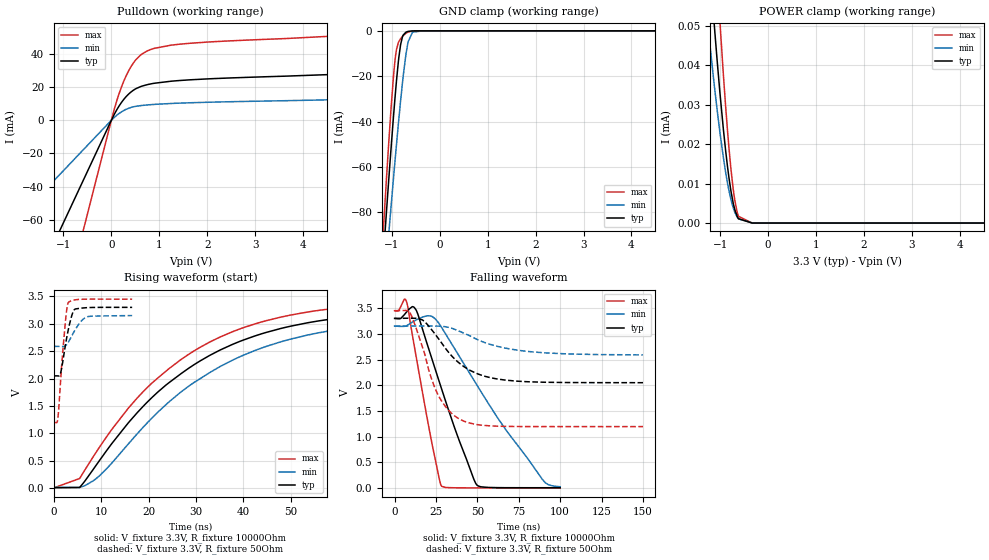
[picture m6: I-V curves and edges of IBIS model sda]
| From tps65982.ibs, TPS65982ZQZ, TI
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|   sda Model
[Model]   sda
Model_type   I/O_open_drain
Polarity   Non-Inverting
Vinl = 0.80
Vinh = 2.00
Vmeas = 1.65
Vref = 3.3
Cref = 2pF
Rref = 10000
|   typ   min   max
|   (nom PVT)   (fast PVT)   (slow PVT)
C_comp   8.631e-13   8.474e-13   8.892e-13
| Where nom  PVT is Nominal Process, 3.3V, 27C
|   Fast PVT is Strong Process,  3.45V, -40C
|   Slow PVT is Weak Process,   3.15V, 125C
[Voltage Range]   3.3   3.15   3.45
|Junction Temperature
[Temperature Range]   27   125   -40
[Pullup Reference]   3.3   3.15   3.45
[Pulldown Reference]   0   0   0
[Power Clamp Reference]   3.3   3.15   3.45
[GND Clamp Reference]   0   0   0
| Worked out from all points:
|   slope of the pulldown table from 0 to 0.495 V, typ, clamps not added: 26.4 ohm
|   GND clamp passes 1 mA (typ) near -0.72 V on its own axis
|   falling waveform, V_fixture 3.3V, R_fixture 10000Ohm: 20-80 % time 20.9ns typ, 38.8ns min, 11.8ns max; typ from 3.3 V to 0.005 V
|   rising waveform, V_fixture 3.3V, R_fixture 10000Ohm: 20-80 % time 26.8ns typ, 28.1ns min, 25.7ns max; typ from 0.005 V to 3.28 V
|   falling waveform, V_fixture 3.3V, R_fixture 50Ohm: 20-80 % time 21.9ns typ, 30.4ns min, 15.2ns max; typ from 3.3 V to 2.05 V
|   rising waveform, V_fixture 3.3V, R_fixture 50Ohm: 20-80 % time 1.6ns typ, 2.37ns min, 1.21ns max; typ from 2.05 V to 3.3 V
[Pulldown]
|   Voltage   I(typ)   I(min)   I(max)
-3.3V     -204.1mA   -100.3mA   -374.1mA
-55.5mV   -3.433mA   -1.687mA   -6.291mA
63.75mV   3.72mA     1.782mA    6.922mA
132.8mV   7.276mA    3.46mA     13.56mA
308.7mV   14.28mA    6.613mA    26.84mA
412.2mV   17.12mA    7.756mA    32.46mA
519.2mV   19.17mA    8.464mA    36.77mA
753.8mV   21.53mA    9.255mA    41.92mA
1.251V    23.57mA    10.13mA    45.33mA
1.645V    24.41mA    10.56mA    46.48mA
5.363V    28.43mA    12.81mA    51.9mA
6.6V      30.96mA    14.1mA     56.05mA
[GND Clamp]
|   Voltage   I(typ)   I(min)   I(max)
-3.3V     -791.8mA   -699.1mA   -889.8mA
-1.224V   -114.3mA   -131mA     -104.8mA
-1.109V   -79.45mA   -101.3mA   -64.81mA
-1.048V   -61.35mA   -85.78mA   -44.54mA
-964.4mV  -38mA      -65.16mA   -20.22mA
-909.2mV  -23.91mA   -51.95mA   -9.276mA
-815.1mV  -6.041mA   -30.79mA   -3.458mA
-704.4mV  -609.6uA   -10.43mA   -1.076mA
-656.7mV  -253.9uA   -4.76mA    -515.7uA
-565.8mV  -41.12uA   -559.3uA   -79.89uA
-330mV    -101.2nA   -940.3nA   -65.96nA
6.6V      0A         0A         0A
[POWER Clamp]
|   Voltage   I(typ)   I(min)   I(max)
-3.3V     548.7uA    403.1uA    721.8uA
-1.299V   79.98uA    55.9uA     116.4uA
-1.208V   64.23uA    44.79uA    94.82uA
-1.111V   48.63uA    33.84uA    73.12uA
-1.004V   33.07uA    23.01uA    51.08uA
-881.5mV  18.07uA    12.69uA    29.13uA
-815.1mV  11.51uA    8.232uA    19.09uA
-774.6mV  8.211uA    6.002uA    13.83uA
-695.3mV  3.499uA    2.796uA    5.93uA
-615.9mV  1.099uA    1.051uA    1.702uA
-330mV    0A         10.54nA    0A
6.6V      0A         0A         0A
[Ramp]
R_load = 10000
|   typ   min   max
dV/dt_r   1.96448/2.68001e-08   1.86582/2.80203e-08   2.05933/2.56579e-08
dV/dt_f   1.97678/2.08968e-08   1.87506/3.88653e-08   2.06819/1.17646e-08
[Falling Waveform]
V_fixture = 3.3V
V_fixture_min = 3.15V
V_fixture_max = 3.45V
R_fixture = 10000Ohm
|   Time   V(typ)   V(min)   V(max)
0s        3.3V       3.15V      3.45V
2.424ns   3.294V     3.145V     3.453V
5.862ns   3.371V     3.145V     3.673V
7.466ns   3.433V     3.162V     3.601V
13.1ns    3.458V     3.27V      2.544V
22.06ns   2.561V     3.344V     951.2mV
28.5ns    1.918V     3.118V     32.31mV
49.65ns   59.37mV    2.006V     3.042mV
89.15ns   5.387mV    171.5mV    3.011mV
100ns     5.367mV    24.9mV     3.011mV
[Rising Waveform]
V_fixture = 3.3V
V_fixture_min = 3.15V
V_fixture_max = 3.45V
R_fixture = 10000Ohm
|   Time   V(typ)   V(min)   V(max)
0s        5.363mV    10.67mV    3.011mV
5.446ns   9.247mV    13.61mV    173.7mV
8.836ns   404.4mV    165.1mV    640.9mV
15.68ns   1.186V     800.5mV    1.453V
20.71ns   1.652V     1.277V     1.917V
26.94ns   2.094V     1.761V     2.352V
35.17ns   2.523V     2.222V     2.761V
44.83ns   2.842V     2.586V     3.057V
55.95ns   3.053V     2.836V     3.246V
90ns      3.279V     3.12V      3.435V
[Falling Waveform]
V_fixture = 3.3V
V_fixture_min = 3.15V
V_fixture_max = 3.45V
R_fixture = 50Ohm
|   Time   V(typ)   V(min)   V(max)
0s        3.3V       3.15V      3.45V
9.342ns   3.303V     3.152V     3.408V
16.79ns   3.271V     3.152V     2.744V
22ns      3.095V     3.151V     2.153V
25.84ns   2.935V     3.15V      1.839V
32.69ns   2.637V     3.124V     1.509V
40.59ns   2.391V     3.03V      1.319V
55.52ns   2.165V     2.817V     1.214V
78.48ns   2.07V      2.664V     1.196V
150ns     2.049V     2.59V      1.195V
[Rising Waveform]
V_fixture = 3.3V
V_fixture_min = 3.15V
V_fixture_max = 3.45V
R_fixture = 50Ohm
|   Time   V(typ)   V(min)   V(max)
0s        2.049V     2.587V     1.195V
870ps     2.047V     2.587V     1.287V
1.418ns   2.098V     2.587V     1.944V
2.202ns   2.48V      2.588V     2.806V
2.73ns    2.749V     2.622V     3.261V
3.064ns   2.895V     2.664V     3.388V
3.802ns   3.154V     2.781V     3.423V
4.524ns   3.269V     2.894V     3.438V
7.212ns   3.296V     3.132V     3.45V
16.54ns   3.3V       3.15V      3.45V
